[IBIS Ver]  4.0
[File Name]  lpc2919_lqfp144.ibs
[File Rev]  1.1
[Date]  Fri Dec 19 10:34:29 2008
[Source]  Package model from Ansoft Q3D Extractor 8.0
[Notes]   IO models Rev 0.20 IBIS Model Design Automation Generation
[Copyright]  NXP Semiconductors 2008. All rights reserved.
[Disclaimer]
| NXP Semiconductors warrants and represents that the IBIS models
| identified herein are owned by NXP Semiconductors (NXP).  The
| models provided are not warranted as fully representing all of the
| operating characteristics and specifications of the semiconductor
| products to which the models relate.  Moreover, unless there is a
| signed, written agreement to the contrary, these models are furnished
| on an "as is" basis without support or warranty of any kind, either
| expressed or implied, regarding the use thereof, and NXP
| specifically disclaims all implied warranties of merchantability and
| fitness of the models for any purpose.
| NXP does not assume any liability arising out of the application
| or use of these IBIS models including infringement of patents and
| copyrights, nor does NXP convey any license under its patents and
| copyrights or the rights of others.
| NXP provides IBIS models as a service to our customers.  You and
| your company shall not distribute, convey, sell, or give these models
| to anyone else without receiving prior written permission from
| NXP.
[Define Package Model]  SOT486EB3
[Manufacturer]  NXP
[OEM]  NXP
[Description]  Simulated @ 100 MHz
[Number Of Pins]  144
[Pin Numbers]
|Pin Num   Terminal Name
1   | diepad:diepad_src
2   | Lead1:Pin1
3   | Lead2:Pin2
4   | Lead3:Pin3
5   | Lead4:Pin4
6   | Lead5:Pin5
7   | Lead6:Pin6
8   | Lead7:Pin7
9   | Lead8:Pin8
10   | Lead9:Pin10
11   | Lead10:Pin12
12   | Lead11:Pin13
13   | Lead12:Pin14
14   | Lead13:Pin15
15   | Lead14:Pin16
16   | Lead15:Pin17
17   | Lead16:Pin18
18   | Lead17:Pin19
19   | Lead18:Pin27
20   | Lead20:Pin29
21   | Lead21:Pin30
22   | Lead22:Pin32
23   | Lead23:Pin34
24   | Lead24:Pin35
25   | Lead25:Pin36
26   | Lead26:Pin39
27   | Lead27:Pin40
28   | Lead28:Pin43
29   | Lead29:Pin45
30   | Lead30:Pin46
31   | Lead31:Pin48
32   | Lead32:Pin49
33   | Lead33:Pin52
34   | Lead34:Pin53
35   | Lead35:Pin54
36   | Lead36:Pin55
37   | Lead37:Pin56
38   | Lead38:Pin57
39   | Lead39:Pin58
40   | Lead40:Pin59
41   | Lead41:Pin60
42   | Lead42:Pin61
43   | Lead43:Pin62
44   | Lead44:Pin64
45   | Lead45:Pin66
46   | Lead46:Pin68
47   | Lead47:Pin72
48   | Lead48:Pin76
49   | Lead49:Pin78
50   | Lead50:Pin82
51   | Lead51:Pin84
52   | Lead52:Pin86
53   | Lead53:Pin88
54   | Lead54:Pin89
55   | Lead55:Pin90
56   | Lead56:Pin91
57   | Lead57:Pin92
58   | Lead58:Pin93
59   | Lead59:Pin94
60   | Lead60:Pin95
61   | Lead61:Pin96
62   | Lead62:Pin97
63   | Lead63:Pin98
64   | Lead64:Pin99
65   | Lead65:Pin100
66   | Lead66:Pin101
67   | Lead67:Pin102
68   | Lead68:Pin103
69   | Lead69:Pin104
70   | Lead70:Pin105
71   | Lead71:Pin106
72   | Lead72:Pin107
73   | Lead73:Pin108
74   | Lead74:Pin109
75   | Lead75:Pin111
76   | Lead76:Pin112
77   | Lead77:Pin113
78   | Lead78:Pin114
79   | Lead79:Pin116
80   | Lead80:Pin117
81   | Lead81:Pin118
82   | Lead82:Pin119
83   | Lead83:Pin120
84   | Lead84:Pin121
85   | Lead85:Pin122
86   | Lead86:Pin123
87   | Lead87:Pin124
88   | Lead88:Pin125
89   | Lead89:Pin127
90   | Lead90:Pin129
91   | Lead91:Pin131
92   | Lead92:Pin132
93   | Lead93:Pin133
94   | Lead94:Pin134
95   | Lead95:Pin136
96   | Lead96:Pin139
97   | Lead97:Pin143
98   | Lead98:Pin145
99   | Lead99:Pin147
100   | Lead100:Pin149
101   | Lead101:Pin154
102   | Lead102:Pin156
103   | Lead103:Pin159
104   | Lead104:Pin161
105   | Lead105:Pin162
106   | Lead106:Pin163
107   | Lead107:Pin164
108   | Lead108:Pin165
109   | Lead109:Pin166
110   | Lead110:Pin167
111   | Lead111:Pin168
112   | Lead112:Pin169
113   | Lead113:Pin170
114   | Lead114:Pin171
115   | Lead115:Pin172
116   | Lead116:Pin173
117   | Lead117:Pin174
118   | Lead118:Pin175
119   | Lead119:Pin178
120   | Lead120:Pin180
121   | Lead121:Pin182
122   | Lead122:Pin184
123   | Lead123:Pin187
124   | Lead124:Pin189
125   | Lead125:Pin191
126   | Lead126:Pin195
127   | Lead127:Pin198
128   | Lead128:Pin199
129   | Lead129:Pin200
130   | Lead130:Pin201
131   | Lead131:Pin202
132   | Lead132:Pin203
133   | Lead133:Pin204
134   | Lead134:Pin205
135   | Lead135:Pin206
136   | Lead136:Pin207
137   | Lead137:Pin208
138   | Lead138:Pin209
139   | Lead139:Pin210
140   | Lead140:Pin211
141   | Lead141:Pin212
142   | Lead142:Pin213
143   | Lead143:Pin214
144   | Lead144:Pin217
[Model Data]
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[End Model Data]
[End Package Model]
[Component]   LPC29XX_LQFP144_01
[Manufacturer]  NXP
[Package]
|[Package Model]  LQFP144
|variable   typ   min   max
R_pkg   0   0   0   |Values included in package model
L_pkg   0   0   0   |Values included in package model
C_pkg   0   0   0   |Values included in package model
| IMPORTANT NOTES:
| This model is valid for the following part types:
| LPC2919/01, LPC2917/01
| Signal names may be slightly different from the data
| sheet due to the 20 Char length limitation
[Pin]   signal_name   model_name   | comments
1 TDO bpats5thpept5v
2 P2.21 bpats5thpept5v
3 P0.24 bpats5thpept5v
4 P0.25 bpats5thpept5v
5 P0.26 bpats5thpept5v
6 P0.27 bpats5thpept5v
7 P0.28 bpats5thpept5v
8 P0.29 bpats5thpept5v
9 POWER_10 POWER
10 P2.22 bpats5thpept5v
11 P2.23 bpats5thpept5v
12 P3.6 bpats5thpept5v
13 P3.7 bpats5thpept5v
14 P0.30 bpats5thpept5v
15 P0.31 bpats5thpept5v
16 P2.24 bpats5thpept5v
17 P2.25 bpats5thpept5v
18 VDD_27 POWER
19 GND_28 POWER
20 P1.31 bpats5thpept5v
21 GNDE_30 POWER
22 P1.30 bpats5thpept5v
23 P3.8 bpats5thpept5v
24 P3.9 bpats5thpept5v
25 P1.29 bpats5thpept5v
26 P1.28 bpats5thpept5v
27 P2.26 bpats5thpept5v
28 P2.27 bpats5thpept5v
29 P1.27 bpats5thpept5v
30 P1.26 bpats5thpept5v
31 POWER_48 POWER
32 P1.25 bpats5thpept5v
33 P1.24 bpats5thpept5v
34 P1.23 bpats5thpept5v
35 P1.22 bpats5thpept5v
36 TMS bpats5thpept5v
37 TCK bpats5thpept5v
38 P1.21 bpats5thpept5v
39 P1.20 bpats5thpept5v
40 P1.19 bpats5thpept5v
41 P1.18 bpats5thpept5v
42 P1.17 bpats5thpept5v
43 GNDE_62 POWER
44 P1.16 bpats5thpept5v
45 P2.0 bpats5thpept5v
46 P2.1 bpats5thpept5v
47 P3.10 bpats5thpept5v
48 P3.11 bpats5thpept5v
49 P1.15 bpats5thpept5v
50 P1.14 bpats5thpept5v
51 P1.13 bpats5thpept5v
52 P1.12 bpats5thpept5v
53 POWER_88 POWER
54 P2.2 bpats5thpept5v
55 P2.3 bpats5thpept5v
56 P1.11 bpats5thpept5v
57 P1.10 bpats5thpept5v
58 P3.12 bpats5thpept5v
59 GND_94 POWER
60 VDD_95 POWER
61 P3.13 bpats5thpept5v
62 P2.4 bpats5thpept5v
63 P2.5 bpats5thpept5v
64 P1.9 bpats5thpept5v
65 GNDE_100 POWER
66 P1.8 bpats5thpept5v
67 P1.7 bpats5thpept5v
68 P1.6 bpats5thpept5v
69 P2.6 bpats5thpept5v
70 P1.5 bpats5thpept5v
71 P1.4 bpats5thpept5v
72 TRSTN bpats5thpept5v
73 RSTN bpats5thpept5v
74 VSSA_OSC POWER
75 XOUT_OSC NC
76 XIN_OSC NC
77 VDDA_OSC POWER
78 VSSA_PLL POWER
79 P2.7 bpats5thpept5v
80 P3.14 bpats5thpept5v
81 P3.15 bpats5thpept5v
82 POWER_119 POWER
83 P2.8 bpats5thpept5v
84 P2.9 bpats5thpept5v
85 P1.3 bpats5thpept5v
86 P1.2 bpats5thpept5v
87 P1.1 bpats5thpept5v
88 GND_125 POWER
89 VDD_127 POWER
90 P1.0 bpats5thpept5v
91 P2.10 bpats5thpept5v
92 P2.11 bpats5thpept5v
93 P0.0 bpats5thpept5v
94 GNDE_134 POWER
95 P0.1 bpats5thpept5v
96 P0.2 bpats5thpept5v
97 P0.3 bpats5thpept5v
98 P3.0 bpats5thpept5v
99 P3.1 bpats5thpept5v
100 P2.12 bpats5thpept5v
101 P2.13 bpats5thpept5v
102 P0.4 bpats5thpept5v
103 P0.5 bpats5thpept5v
104 POWER_161 POWER
105 P0.6 bpats5thpept5v
106 P0.7 bpats5thpept5v
107 A3V3 POWER
108 JTAGSEL bpats5thpept5v
109 A5V POWER
110 VREFP NC
111 VREFN NC
112 P0.8 bpats5thpept5v
113 P0.9 bpats5thpept5v
114 P0.10 bpats5thpept5v
115 P0.11 bpats5thpept5v
116 P2.14 bpats5thpept5v
117 P2.15 bpats5thpept5v
118 P3.2 bpats5thpept5v
119 GNDE_178 POWER
120 P3.3 bpats5thpept5v
121 P0.12 bpats5thpept5v
122 P0.13 bpats5thpept5v
123 P0.14 bpats5thpept5v
124 P0.15 bpats5thpept5v
125 P0.16 bpats5thpept5v
126 P0.17 bpats5thpept5v
127 VDD_198 POWER
128 GND_199 POWER
129 P2.16 bpats5thpept5v
130 P2.17 bpats5thpept5v
131 POWER_202 POWER
132 P0.18 bpats5thpept5v
133 P0.19 bpats5thpept5v
134 P3.4 bpats5thpept5v
135 P3.5 bpats5thpept5v
136 P2.18 bpats5thpept5v
137 P2.19 bpats5thpept5v
138 P0.20 bpats5thpept5v
139 P0.21 bpats5thpept5v
140 P0.22 bpats5thpept5v
141 GNDE_212 POWER
142 P0.23 bpats5thpept5v
143 P2.20 bpats5thpept5v
144 TDI bpats5thpept5v
[Model Selector] bpats5thpept5v
bpats5thpept5v_p   Plain input Mode (p1=0, p2=1)
bpats5thpept5v_pd   Pull Down Mode   (p1=0, p2=0)
bpats5thpept5v_pu   Pull up   Mode   (p1=1, p2=1)
bpats5thpept5v_r   Repeater  Mode   (p1=1, p2=0)
[Model Selector] bpts5ptpht5v
bpts5ptpht5v_p_sh   Plain input Mode (p1=0, p2=1)
bpts5ptpht5v_p_sl   Plain input Mode (p1=0, p2=1)
bpts5ptpht5v_pd_sh   Pull Down Mode (p1=1, p2=1)
bpts5ptpht5v_pd_sl   Pull Down Mode (p1=1, p2=1)
bpts5ptpht5v_pu_sh   Pull Up Mode (p1=0, p2=0)
bpts5ptpht5v_pu_sl   Pull Up Mode (p1=0, p2=0)
bpts5ptpht5v_r_sh   Repeater Mode (p1=1, p2=0)
bpts5ptpht5v_r_sl   Repeater Mode (p1=1, p2=0)
| Models and submodels in the file (16): usb11f1_iom_hs (I/O), usb11f1_iom_ls (I/O), usb11f1_iop_hs (I/O), usb11f1_iop_ls (I/O), bpats5thpept5v_p (I/O), bpats5thpept5v_pd (I/O), bpats5thpept5v_pu (I/O), bpats5thpept5v_r (I/O), bpts5ptpht5v_p_sh (I/O), bpts5ptpht5v_p_sl (I/O), bpts5ptpht5v_pd_sh (I/O), bpts5ptpht5v_pd_sl (I/O), bpts5ptpht5v_pu_sh (I/O), bpts5ptpht5v_pu_sl (I/O), bpts5ptpht5v_r_sh (I/O), bpts5ptpht5v_r_sl (I/O)
